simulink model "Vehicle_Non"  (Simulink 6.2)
settings: Solver=ode45  StartTime=0.0  StopTime=1000  FixedStep=Ts  RelTol=1e-3
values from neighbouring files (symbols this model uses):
  Ave = [    [vehicle_flex34.m]    (also in vehicle_rigid.m)
  Bve = [    [vehicle_flex34.m]    (also in vehicle_rigid.m)
  CB2L = [cpsi, -cphi*spsi,  sphi*spsi;          0,    cphi,      -sphi;          0,    sphi*cpsi,  cphi*cpsi]/cpsi    [Rigbod_Dynam_LVLH.m]    (also in start.m = eye(3); start2.m = eye(3); start3.m = eye(3); start1.m = eye(3))
  Cve = [    [vehicle_flex34.m]    (also in vehicle_rigid.m)
  Dve = [    [vehicle_flex34.m]    (also in vehicle_rigid.m)
  ini = [wbo; atto; Hco]    [start.m]    (also in start2.m; start3.m; start1.m)
  nt = 12    [start.m]    (also in start2.m; start3.m; start1.m)
  wo = 0.0011    [start.m]    (also in start2.m; start3.m; start1.m)
undefined symbols (not defined in the file or in its folder): Rigbod_Dynam_LVLH

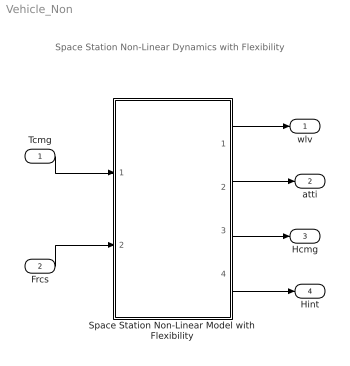
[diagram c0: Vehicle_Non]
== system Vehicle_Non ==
  note: Space Station Non-Linear Dynamics with Flexibility
  Tcmg : Inport  Port=1  LatchInput=off
  Frcs : Inport  Port=2  LatchInput=off
  Space Station Non-Linear Model with Flexibility : Subsystem
  wlv : Outport
  atti : Outport  Port=2
  Hcmg : Outport  Port=3
  Hint : Outport  Port=4
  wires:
  Tcmg/1 -> Space Station Non-Linear Model with Flexibility/1(Tcmg)
  Space Station Non-Linear Model with Flexibility/1(wlv) -> wlv/1
  Frcs/1 -> Space Station Non-Linear Model with Flexibility/2(Frcs)
  Space Station Non-Linear Model with Flexibility/2(atti) -> atti/1
  Space Station Non-Linear Model with Flexibility/4(Hint) -> Hint/1
  Space Station Non-Linear Model with Flexibility/3(Hcmg) -> Hcmg/1

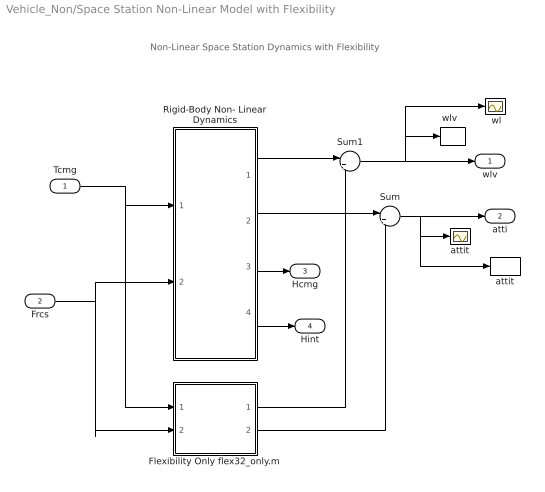
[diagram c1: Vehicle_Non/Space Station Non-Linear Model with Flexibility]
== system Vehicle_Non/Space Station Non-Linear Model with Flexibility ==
  note: Non-Linear Space Station Dynamics with Flexibility
  Tcmg : Inport  Port=1  LatchInput=off
  Frcs : Inport  Port=2  LatchInput=off
  " attit " : Scope
  " wl" : Scope
  Flexibility Only flex32_only.m : Subsystem
  Rigid-Body Non- Linear Dynamics : Subsystem
  Sum : Sum  Inputs=|++
  Sum1 : Sum  Inputs=|++
  attit : ToWorkspace  VariableName=atti  SampleTime=-1  SaveFormat=Array
  "wlv  " : ToWorkspace  VariableName=wl  SampleTime=-1  SaveFormat=Array
  wlv : Outport
  atti : Outport  Port=2
  Hcmg : Outport  Port=3
  Hint : Outport  Port=4
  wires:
  Frcs/1 -> Rigid-Body Non- Linear Dynamics/2(Frcs), Flexibility Only flex32_only.m/2(Frcs)
  Rigid-Body Non- Linear Dynamics/2(atti-lv) -> Sum/1
  Flexibility Only flex32_only.m/2(att) -> Sum/2
  Sum/1 -> atti/1, " attit "/1, attit/1
  Sum1/1 -> wlv/1, "wlv  "/1, " wl"/1
  Tcmg/1 -> Rigid-Body Non- Linear Dynamics/1(Tcmg), Flexibility Only flex32_only.m/1(Tcmg)
  Rigid-Body Non- Linear Dynamics/1(w-lv) -> Sum1/1
  Flexibility Only flex32_only.m/1(wbf) -> Sum1/2
  Rigid-Body Non- Linear Dynamics/3(Hcmg) -> Hcmg/1
  Rigid-Body Non- Linear Dynamics/4(Hint) -> Hint/1

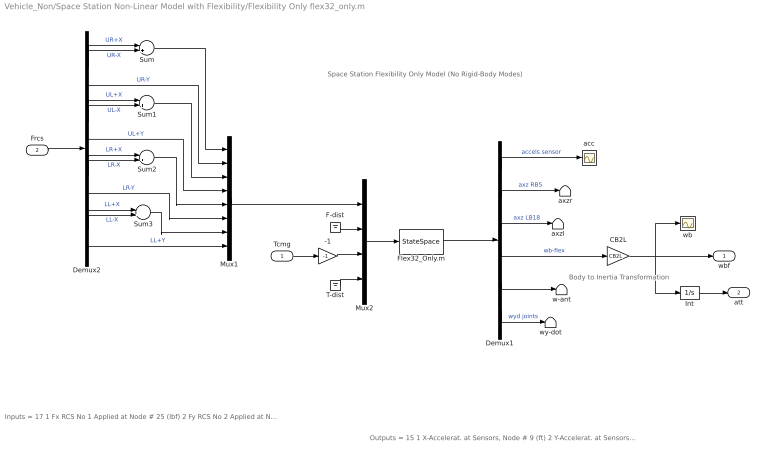
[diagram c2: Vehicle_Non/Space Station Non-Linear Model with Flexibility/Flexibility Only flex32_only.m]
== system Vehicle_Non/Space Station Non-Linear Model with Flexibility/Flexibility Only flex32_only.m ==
  note: Outputs = 15 1 X-Accelerat. at Sensors, Node # 9 (ft) 2 Y-Accelerat. at Sensors, Node # 9 (ft) 3 Z-Accelerat. at Sensors, Node # 9 (ft) 4 X-Accelerat. at Right Boom End, Node # 5 (ft) 5 Z-Accelerat. at Right Boom End, Node # 5 (ft) 6 X-Accelerat. at Left Boom End, Node # 18 (ft) 7 Z-Accelerat. at Left Boom End, Node # 18 (ft) 8 X-Rot. Rate at Sensors, Node # 9 (radian) 9 Y-Rot. Rate at Sensors, Node # 9 (radian) 10 Z-Rot. Rate at Sensors, Node # 9 (radian) 11 X-Rot. Rate at Antena Bot-Left, Node # 24 (radian) 12 Y-Rot. Rate at Antena Bot-Left, Node # 24 (radian) 13 Z-Rot. Rate at Antena Bot-Left, Node # 24 (radian) 14 Y-Rot.Accel. at Right Joint, Node # 7 (radian) 15 Y-Rot.Accel. at Left Joint, Node # 16 (radian)
  note: Inputs = 17 1 Fx RCS No 1 Applied at Node # 25 (lbf) 2 Fy RCS No 2 Applied at Node # 25 (lbf) 3 Fx RCS No 3 Applied at Node # 26 (lbf) 4 Fy RCS No 4 Applied at Node # 26 (lbf) 5 Fx RCS No 5 Applied at Node # 27 (lbf) 6 Fy RCS No 6 Applied at Node # 27 (lbf) 7 Fx RCS No 7 Applied at Node # 28 (lbf) 8 Fy RCS No 8 Applied at Node # 28 (lbf) 9 Fx Disturb. No 9 at Node # 21 (lbf) 10 Fy Disturb. No 10 at Node # 21 (lbf) 11 Fz Disturb. No 11 at Node # 21 (lbf) 12 Torq-x No 1 CMG Applied at Node # 10 (ft-lb) 13 Torq-y No 2 CMG Applied at Node # 10 (ft-lb) 14 Torq-z No 3 CMG Applied at Node # 10 (ft-lb) 15 Torq-x No 4 Gimbal Dist. at Node # 1 (ft-lb) 16 Torq-y No 5 Gimbal Dist. at Node # 1 (ft-lb) 17 Torq-z No 6 Gimbal Dist. at Node # 1 (ft-lb)
  note: Space Station Flexibility Only Model (No Rigid-Body Modes)
  note: Body to Inertia Transformation
  Tcmg : Inport  Port=1  LatchInput=off
  Frcs : Inport  Port=2  LatchInput=off
  -1 : Gain  Gain=-1
  CB2L : Gain  Gain=CB2L  Multiplication=Matrix(K*u)
  Demux1 : Demux  Outputs=[3, 2, 2, 3, 3, 2]
  Demux2 : Demux  Outputs=12
  F-dist : Ground
  Flex32_Only.m : StateSpace  A=Ave  B=Bve  C=Cve  D=Dve
  Int : Integrator
  Mux1 : Mux  Inputs=8
  Mux2 : Mux  Inputs=[8, 3, 3, 3]
  Sum{,1..3} (4 alike) : Sum  Inputs=|+-
  T-dist : Ground
  acc : Scope
  axzl : Terminator
  axzr : Terminator
  w-ant : Terminator
  wb : Scope
  wy-dot : Terminator
  wbf : Outport
  att : Outport  Port=2
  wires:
  Demux1/6 -> wy-dot/1  "wyd joints"
  Demux1/5 -> w-ant/1
  T-dist/1 -> Mux2/4
  F-dist/1 -> Mux2/2
  Demux1/3 -> axzl/1  "axz LB18"
  Demux1/2 -> axzr/1  "axz RB5"
  Tcmg/1 -> -1/1
  Demux1/4 -> CB2L/1  "wb-flex"
  Demux1/1 -> acc/1  "accels sensor"
  Flex32_Only.m/1 -> Demux1/1
  Mux2/1 -> Flex32_Only.m/1
  Mux1/1 -> Mux2/1
  Frcs/1 -> Demux2/1
  Demux2/6 -> Mux1/4  "UL+Y"
  Demux2/9 -> Mux1/6  "LR-Y"
  Demux2/12 -> Mux1/8  "LL+Y"
  Demux2/3 -> Mux1/2  "UR-Y"
  Demux2/1 -> Sum/1  "UR+X"
  Demux2/2 -> Sum/2  "UR-X"
  Sum/1 -> Mux1/1
  Demux2/4 -> Sum1/1  "UL+X"
  Demux2/5 -> Sum1/2  "UL-X"
  Sum1/1 -> Mux1/3
  Demux2/7 -> Sum2/1  "LR+X"
  Demux2/8 -> Sum2/2  "LR-X"
  Demux2/10 -> Sum3/1  "LL+X"
  Demux2/11 -> Sum3/2  "LL-X"
  Sum3/1 -> Mux1/7
  Sum2/1 -> Mux1/5
  Int/1 -> att/1
  -1/1 -> Mux2/3
  CB2L/1 -> wb/1, wbf/1, Int/1

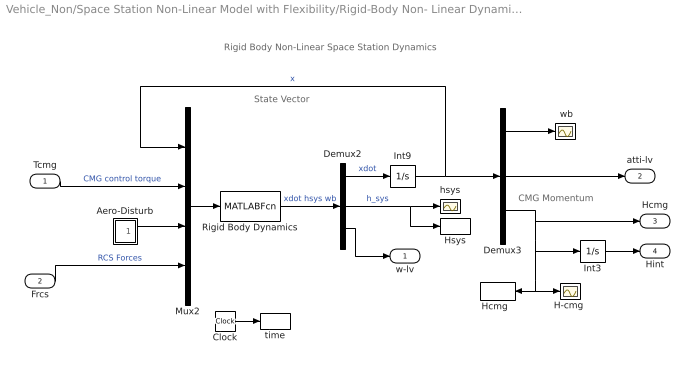
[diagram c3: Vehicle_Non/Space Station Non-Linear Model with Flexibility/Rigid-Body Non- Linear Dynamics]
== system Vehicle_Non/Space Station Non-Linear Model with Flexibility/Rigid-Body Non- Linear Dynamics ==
  note: CMG Momentum
  note: State Vector
  note: Rigid Body Non-Linear Space Station Dynamics
  Tcmg : Inport  Port=1  PortDimensions=3  LatchInput=off
  Frcs : Inport  Port=2  PortDimensions=nt  LatchInput=off
  " wb" : Scope
  Aero-Disturb : Subsystem
  Clock : Clock
  Demux2 : Demux  Outputs=[9,3,3]
  Demux3 : Demux  Outputs=[3,3,3]
  "H-cmg " : Scope
  "Hcmg  " : ToWorkspace  VariableName=Hcmg  SampleTime=-1  SaveFormat=Array
  Hsys : ToWorkspace  VariableName=Hsys  SampleTime=-1  SaveFormat=Array
  Int3 : Integrator
  Int9 : Integrator  InitialCondition=ini
  Mux2 : Mux  Inputs=[9, 3, 3, nt]
  Rigid Body Dynamics : MATLABFcn  MATLABFcn=Rigbod_Dynam_LVLH( u(1:9), u(10:12), u(13:15), u(16:15+nt) )  OutputDimensions=15
  hsys : Scope
  time : ToWorkspace  VariableName=time  SampleTime=-1  SaveFormat=Array
  w-lv : Outport
  atti-lv : Outport  Port=2
  Hcmg : Outport  Port=3
  Hint : Outport  Port=4
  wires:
  Mux2/1 -> Rigid Body Dynamics/1
  Clock/1 -> time/1
  Frcs/1 -> Mux2/4  "RCS Forces"
  Demux3/3 -> Hcmg/1, "H-cmg "/1, "Hcmg  "/1, Int3/1
  Demux3/2 -> atti-lv/1
  Demux2/2 -> Hsys/1, hsys/1  "h_sys"
  Demux2/3 -> w-lv/1
  Tcmg/1 -> Mux2/2  "CMG control torque"
  Int9/1 -> Mux2/1, Demux3/1  "x"
  Demux2/1 -> Int9/1  "xdot"
  Rigid Body Dynamics/1 -> Demux2/1  "xdot hsys wb"
  Demux3/1 -> " wb"/1
  Aero-Disturb/1(Td) -> Mux2/3
  Int3/1 -> Hint/1

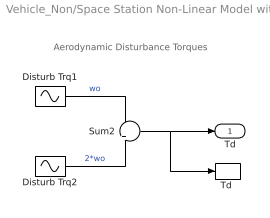
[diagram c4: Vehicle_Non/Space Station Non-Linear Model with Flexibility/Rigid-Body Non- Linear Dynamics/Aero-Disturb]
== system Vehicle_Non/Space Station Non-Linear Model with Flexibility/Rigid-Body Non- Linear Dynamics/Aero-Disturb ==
  note: Aerodynamic Disturbance Torques
  Disturb Trq1 : Sin  Amplitude=[1, 3, 1]  Bias="[1  8  1]"  Frequency=[wo, wo, wo]  SampleTime=0
  Disturb Trq2 : Sin  Amplitude=[1, 1, 1]*0.5  Frequency=[wo, wo, wo]*2  SampleTime=0
  Sum2 : Sum  Inputs=+|+
  "Td " : ToWorkspace  VariableName=Td  SampleTime=-1  SaveFormat=Array
  Td : Outport
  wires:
  Disturb Trq2/1 -> Sum2/2  "2*wo"
  Sum2/1 -> "Td "/1, Td/1
  Disturb Trq1/1 -> Sum2/1  "wo"
